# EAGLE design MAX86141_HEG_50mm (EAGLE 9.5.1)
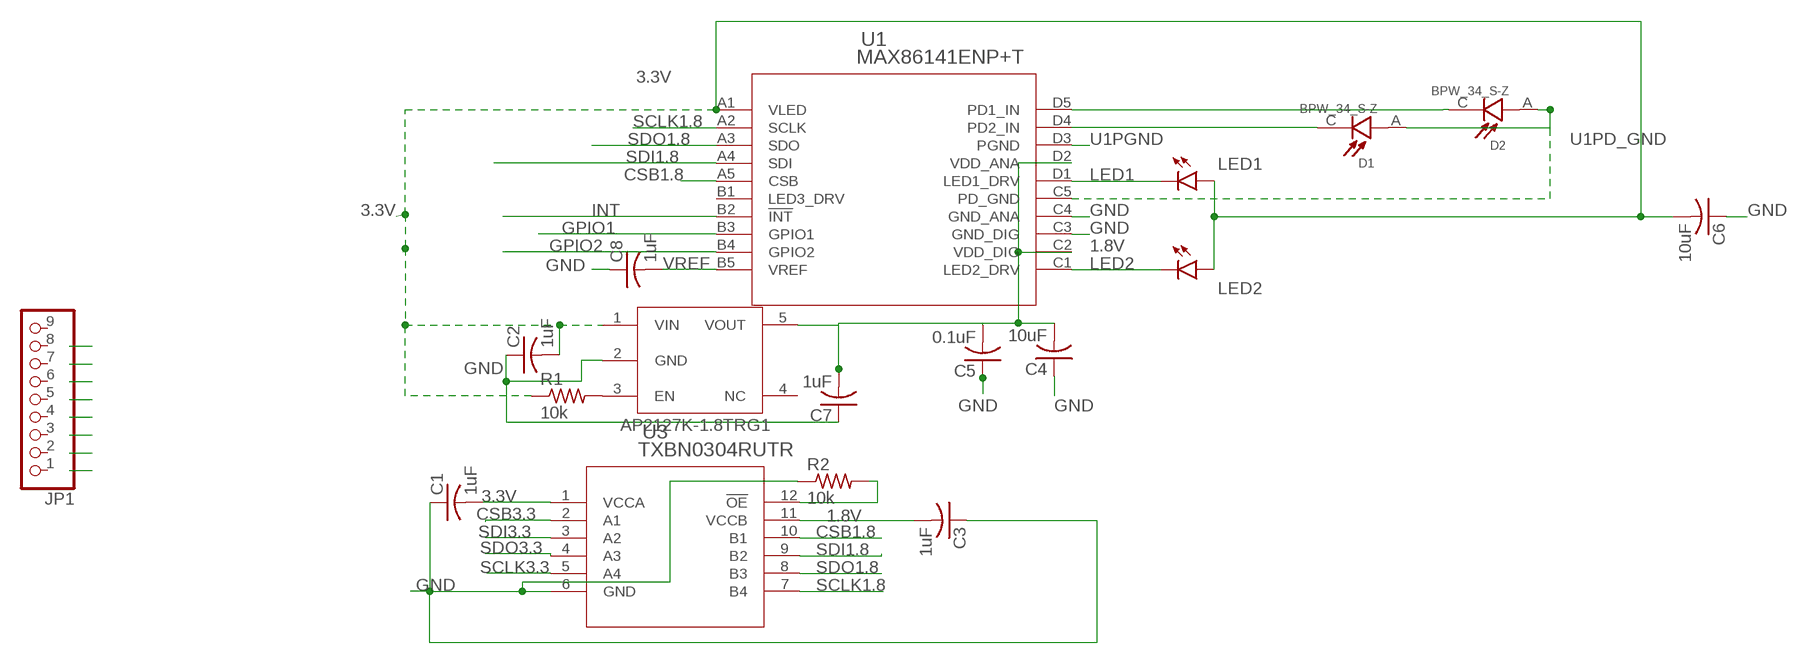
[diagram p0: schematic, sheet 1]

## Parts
C1  1uF  C-USC0402  [C0402]
C2  1uF  C-USC0402  [C0402]
C3  1uF  C-USC0402  [C0402]
C4  10uF  C-USC0402  [C0402]
C5  0.1uF  C-USC0402  [C0402]
C6  10uF  C-USC0402  [C0402]
C7  1uF  C-USC0402  [C0402]
C8  1uF  C-USC0402  [C0402]
D1  BPW_34_S-Z  [DIO_BPW_34_S-Z]
D2  BPW_34_S-Z  [DIO_BPW_34_S-Z]
JP1  PINHD-1X9  [1X09]
LED1  LEDCHIPLED_1206  [CHIPLED_1206]
LED2  LEDCHIPLED_1206  [CHIPLED_1206]
R1  10k  R-US_R0402  [R0402]
R2  10k  R-US_R0402  [R0402]
U1  MAX86141ENP+T  [21-100134A_20]
U2  AP2127K-1.8TRG1  [SOT23-5L]
U3  TXBN0304RUTR  [RUT12]

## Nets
1.8V: C3.2 C4.2 C5.2 C7.2 U1.C2(VDD_DIG) U1.D2(VDD_ANA) U2.5(VOUT) U3.11(VCCB)
3.3V: C1.2 C2.2 C6.2 LED1.A LED2.A R1.1 U1.A1(VLED) U2.1(VIN) U3.1(VCCA)
CSB1.8: U1.A5(CSB) U3.10(B1)
CSB3.3: U3.2(A1)
GND: C1.1 C2.1 C3.1 C4.1 C5.1 C6.1 C7.1 C8.1 R2.1 U1.C3(GND_DIG) U1.C4(GND_ANA) U2.2(GND) U3.6(GND)
GPIO1: U1.B3(GPIO1)
GPIO2: U1.B4(GPIO2)
INT: U1.B2(!INT)
LED1: LED1.C U1.D1(LED1_DRV)
LED2: LED2.C U1.C1(LED2_DRV)
N$1: R1.2 U2.3(EN)
OE: R2.2 U3.12(!OE)
PD1_IN: D2.C U1.D5(PD1_IN)
PD2_IN: D1.C U1.D4(PD2_IN)
SCLK1.8: U1.A2(SCLK) U3.7(B4)
SCLK3.3: U3.5(A4)
SDI1.8: U1.A4(SDI) U3.9(B2)
SDI3.3: U3.3(A2)
SDO1.8: U1.A3(SDO) U3.8(B3)
SDO3.3: U3.4(A3)
U1PD_GND: D1.A D2.A U1.C5(PD_GND)
U1PGND: U1.D3(PGND)
VREF: C8.2 U1.B5(VREF)
Unconnected: JP1.1 JP1.2 JP1.3 JP1.4 JP1.5 JP1.6 JP1.7 JP1.8 JP1.9 U1.B1(LED3_DRV) U2.4(NC)

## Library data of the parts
C1-C8 = adafruit:C-US: CAPACITOR, American symbol
D1 D2 = BPW_34_S-Z:BPW_34_S-Z: Silicon PIN Photodiode; DESCRIPTION: Photodiode 850nm 20ns 120° 2-SMD, Gull Wing; DIGI-KEY_PART_NUMBER: 475-2659-1-ND; DIGI-KEY_PURCHASE_URL: https://www.digikey.com/product-detail/en/osram-opto-semiconductors-inc/BPW-34-S-Z/475-2659-1-ND/1893861?utm_source=snapeda&utm_medium=aggregator&utm_campaign=symbol; MF: OSRAM Opto; MP: BPW 34 S-Z; PACKAGE: SMD-2 OSRAM Opto
JP1 = pinhead:PINHD-1X9: PIN HEADER
LED1 LED2 = led:LED: LED
R1 R2 = adafruit:R-US_: RESISTOR, American symbol
U1 = MAX86141:MAX86141ENP+T; MANUFACTURER_PART_NUMBER: MAX86141ENP+T; VENDOR: Maxim Integrated Products
U2 = AP2127K:AP2127K-1.8TRG1
U3 = TXBN0304:TXBN0304RUTR; BUILT_BY: EMA_UL_Team; MANUFACTURER_PART_NUMBER: TXBN0304RUTR; VENDOR: Texas Instruments

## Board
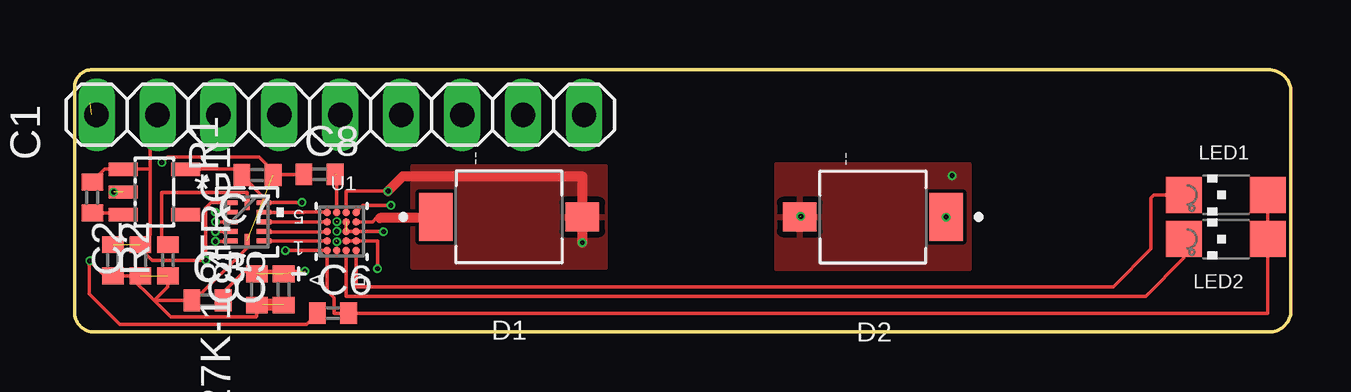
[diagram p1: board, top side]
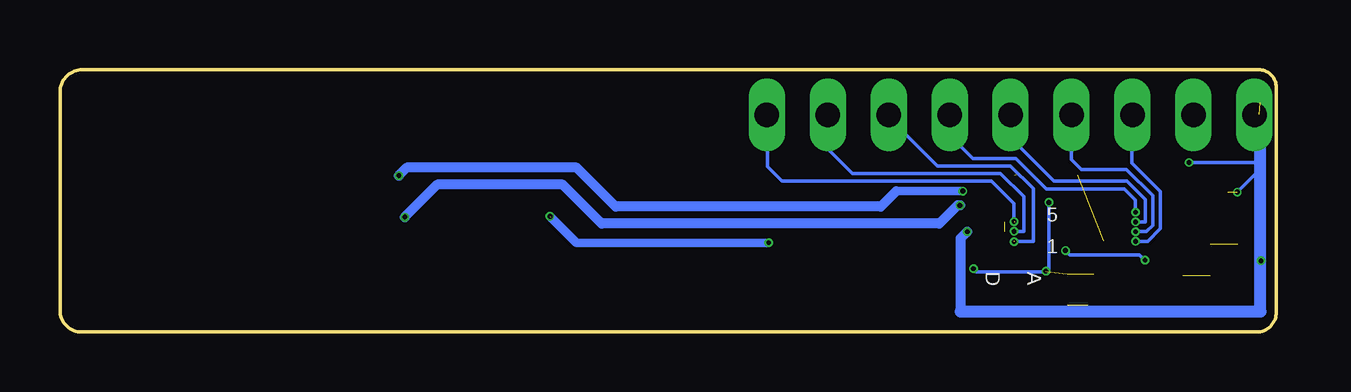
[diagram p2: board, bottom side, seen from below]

Size 50.7 x 10.95 mm. Coordinates in mm from the lower left corner, seen from the top.
Outline: 49.78,0 arc90 50.7,0.91 50.7,10.01 arc90 49.76,10.95 0.74,10.95 arc90 0,10.21 0,0.84 arc90 0.81,0 49.78,0
Copper layers (1*16): Top 0.035mm / dielectric 1.5mm / Bottom 0.035mm
Design rules "default *": minimum track width 6mil, minimum drill 0.35mm, track to track 6mil, track to pad 6mil, pad to pad 6mil, via to via 2mil, smd to smd 6mil, copper to edge 40mil, drill to drill 6mil, minimum pad ring 10mil, minimum via ring 3mil, stop-mask expansion 4mil, vias tented up to drill 0mil, thermal gap 10mil

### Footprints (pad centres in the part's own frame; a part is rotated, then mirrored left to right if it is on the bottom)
C0402 = smd 0.7 x 0.9: 1 -0.65,0; 2 0.65,0
DIO_BPW_34_S-Z = smd 1.4 x 1.2: A -3.05,0 | smd 1.4 x 2: C 3.05,0
1X09 = drill 1.016 long: 1 -10.16,0; 2 -7.62,0; 3 -5.08,0; 4 -2.54,0; 5 0,0; 6 2.54,0; 7 5.08,0; 8 7.62,0; 9 10.16,0
CHIPLED_1206 = smd 1.5 x 1.5: A 0,-1.75; C 0,1.75
R0402 = smd 0.7 x 0.9: 1 -0.65,0; 2 0.65,0
21-100134A_20 = smd 0.305 x 0.305: A1 -0.8,0.6; A2 -0.4,0.6; A3 0,0.6; A4 0.4,0.6; A5 0.8,0.6; B1 -0.8,0.2; B2 -0.4,0.2; B3 0,0.2; B4 0.4,0.2; B5 0.8,0.2; C1 -0.8,-0.2; C2 -0.4,-0.2; C3 0,-0.2; C4 0.4,-0.2; C5 0.8,-0.2; D1 -0.8,-0.6; D2 -0.4,-0.6; D3 0,-0.6; D4 0.4,-0.6; D5 0.8,-0.6
SOT23-5L = smd 0.55 x 1.2: 1 -0.95,-1.3; 2 0,-1.3; 3 0.95,-1.3; 4 0.95,1.3; 5 -0.95,1.3
RUT12 = smd 0.6 x 0.2: 1 -0.7,0.8; 2 -0.7,0.4; 3 -0.7,0; 4 -0.7,-0.4; 5 -0.7,-0.8; 7 0.7,-0.8; 8 0.7,-0.4; 9 0.7,0; 10 0.7,0.4; 11 0.7,0.8 | smd 0.2 x 0.6: 6 0,-0.8; 12 0,0.8

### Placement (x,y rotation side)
C1  1.6,3 90 top
C2  2.74,3 90 top
C3  5.54,1.32 0 top
C4  7.59,1.78 90 top
C5  8.71,1.78 90 top
C6  10.77,0.79 0 top
C7  7.62,6.55 180 top
C8  10.21,6.58 0 top
D1  18.11,4.8 180 top
D2  33.27,4.8 0 top
JP1  11.07,9.07 0 top
LED1  47.99,5.72 90 top
LED2  47.99,3.88 90 top
R1  0.74,5.61 270 top
R2  3.89,3 90 top
U1  11.13,4.2 90 top
U2  3.33,5.84 270 top
U3  7.19,4.6 0 top

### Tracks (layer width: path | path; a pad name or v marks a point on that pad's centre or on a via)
1.8V  (via drill 0.2)  (2 unrouted)
  Top 0.152: U1.C2 U1.D2 12.62,3.8 v12.62,2.64 | v9.47,5.41 9.46,5.4 U3.11 7.89,5.62 6.95,6.55 | C3.2 6.19,1.67 7.06,2.54 v9.6,2.54 | U2.5 6.72,6.79 6.95,6.55 | C7.2 6.95,6.55
  Bottom 0.152: v12.62,2.64 12.5,2.52 9.47,2.52 9.47,2.54 | 9.47,2.54 v9.6,2.54 | v9.47,5.41 9.47,2.54
3.3V  (via drill 0.2)  (1 unrouted)
  Top 0.152: LED1.A LED2.A 49.74,0.79 C6.2 10.83,0.79 10.83,1.43 10.53,1.73 U1.A1 | 3.15,9.02 3.15,6.79 | U1.A1 10.53,1.75 | v8.79,3.4 U1.A1 | 3.15,6.79 U2.1 1.27,6.79 R1.1 | 3.15,6.79 3.15,4.05 C2.2 2.74,3.5 3.24,3 v5.47,3 5.47,5.18 5.69,5.4 U3.1
  Bottom 0.152: v5.47,3 5.7,3.23 8.61,3.23 v8.79,3.4
CSB1.8
  Top 0.152: U1.A5 9.55,5 U3.10
CSB3.3  (via drill 0.2)
  Top 0.152: U3.2 v5.87,5
  Bottom 0.152: v5.87,5 5.87,5.51 6.32,5.97 9.58,5.97 10.85,7.24 12.65,7.24 13.61,8.2 13.61,9.09
GND  (via drill 0.2)  (6 unrouted)
  Top 0.152: C8.1 8.41,6.58 8.27,6.72 | 8.27,6.72 7.68,7.3 3.89,7.3 3.66,7.07 v3.63,7.07 | U1.C4 U1.C3 v12.88,4.19 | U3.6 7.19,3.52 4.99,1.32 C3.1 3.31,1.32 | 3.31,1.32 2.29,2.35 C1.1 1.26,2.35 v0.64,2.97 0.61,2.95 0.61,1.6 1.88,0.33 9.66,0.33 C6.1 | 3.31,1.32 4,0.64 7.57,0.64 7.59,0.66 C4.1 7.61,1.14 8.94,1.14 | C7.1 8.27,6.72 | R2.1 3.89,1.9 3.31,1.32
  Top 0.508: 8.94,1.14 7.85,1.14 | C4.1 7.59,1.07
  Bottom 0.152: v3.63,7.07 0.71,7.07 | 0.71,7.07 0.71,9.07 | v1.63,5.84 0.71,6.76 0.71,7.07
  Bottom 0.406: v12.88,4.19 13.16,3.91 13.16,0.86
  Bottom 0.508: 13.16,0.86 0.66,0.86 0.66,9.58
GPIO1  (via drill 0.2)
  Bottom 0.152: U1.B3 10.53,4.2 10.53,5.65 11.49,6.62 17.67,6.62 18.67,7.62 18.67,9.04
  other vias: 10.93,4.2
GPIO2  (via drill 0.2)  (1 unrouted)
  Bottom 0.152: v10.93,4.61 v10.93,4.62 10.93,5.37 11.87,6.31 20.61,6.31 21.21,6.91 21.21,9.04
INT  (via drill 0.2)  (1 unrouted)
  Bottom 0.152: v10.93,3.77 10.91,3.79 10.13,3.79 10.13,5.99 11.07,6.93 14.12,6.93 16.21,9.02
LED1
  Top 0.152: 45.91,5.72 LED1.C 44.99,5.72 44.87,5.59 44.87,3.46 43.29,1.89 11.73,1.89 U1.D1
LED2
  Top 0.152: 45.97,3.88 LED2.C 46.24,3.08 44.65,1.5 11.33,1.5 U1.C1
N$1
  Top 0.152: U2.3 1.96,4.96 R1.2
OE
  Top 0.152: R2.2 3.62,3.91 3.62,5.82 7.19,5.82 U3.12
PD1_IN  (via drill 0.2)
  Top 0.152: U1.D5 12.01,5.28 v13.18,5.28
  Bottom 0.406: v13.18,5.28 13.28,5.28 14.05,4.52 28.12,4.52 29.74,6.15 34.98,6.15 D2.C
  other vias: 36.32,4.8
PD2_IN
  Top 0.152: U1.D4 12.42,4.6 12.57,4.75 12.72,4.75
  Top 0.406: D1.C 15.06,4.75 12.72,4.75
SCLK1.8
  Top 0.152: U1.A2 8.48,3.8 U3.7 7.87,3.79 U3.7
SCLK3.3  (via drill 0.2)
  Top 0.152: U3.5 6.48,3.79 v5.87,3.79
  Bottom 0.152: v5.87,3.79 5.36,3.79 4.83,4.32 4.83,5.87 6.02,7.06 6.02,9.09
SDI1.8
  Top 0.152: U1.A4 9.66,4.6 | 9.66,4.6 | 9.66,4.6 9.28,4.6 U3.9
SDI3.3  (via drill 0.2)
  Top 0.152: U3.3 v5.87,4.6
  Bottom 0.152: v5.87,4.6 5.46,4.6 5.46,5.54 6.22,6.3 9.27,6.3 11.05,8.08 11.05,9.09
SDO1.8
  Top 0.152: U1.A3 10.5,4.17 9.58,4.17 | 9.58,4.17 9.58,4.18 | 9.58,4.17 7.91,4.17 U3.8
SDO3.3  (via drill 0.2)
  Top 0.152: U3.4 v5.87,4.19
  Bottom 0.152: v5.87,4.19 5.41,4.19 5.16,4.45 5.16,5.69 6.25,6.78 8.13,6.78 8.53,7.19 8.53,9.09
U1PD_GND  (via drill 0.2)  (1 unrouted)
  Top 0.152: v13.07,5.88 11.33,5.88 U1.C5
  Top 0.406: v13.07,5.88 13.69,6.5 21.16,6.5 D1.A v21.16,3.73
  Bottom 0.356: 15.84,5.88 v13.07,5.88 | v30.27,4.83 29.18,3.73 v21.16,3.73 21.21,3.73
  Bottom 0.406: 15.84,5.88 16.48,5.23 27.53,5.23 29.16,6.86 36.25,6.86 v36.58,6.53
  pour Top: 14.07,2.67 14.07,6.93 22.15,6.93 22.15,2.67
  pour Top: 29.24,2.62 29.24,7.01 37.31,7.01 37.31,2.62
VREF  (1 unrouted)
  Top 0.152: U1.B5 10.93,6.55

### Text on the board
tPlace: -- | --
tValuesAlt: C7 | C8 | MAX86141 HEG MINI Prototype (MIT License) / Designed By: Joshua Brewster / Sponsored By: Blueberry nIRS Project | LED1 | U2 | R1 | U3 | P2 | P1 | cathode | C3 | U1 | LED2 | C1 | C2 | R2 | C5 | C6 | C4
